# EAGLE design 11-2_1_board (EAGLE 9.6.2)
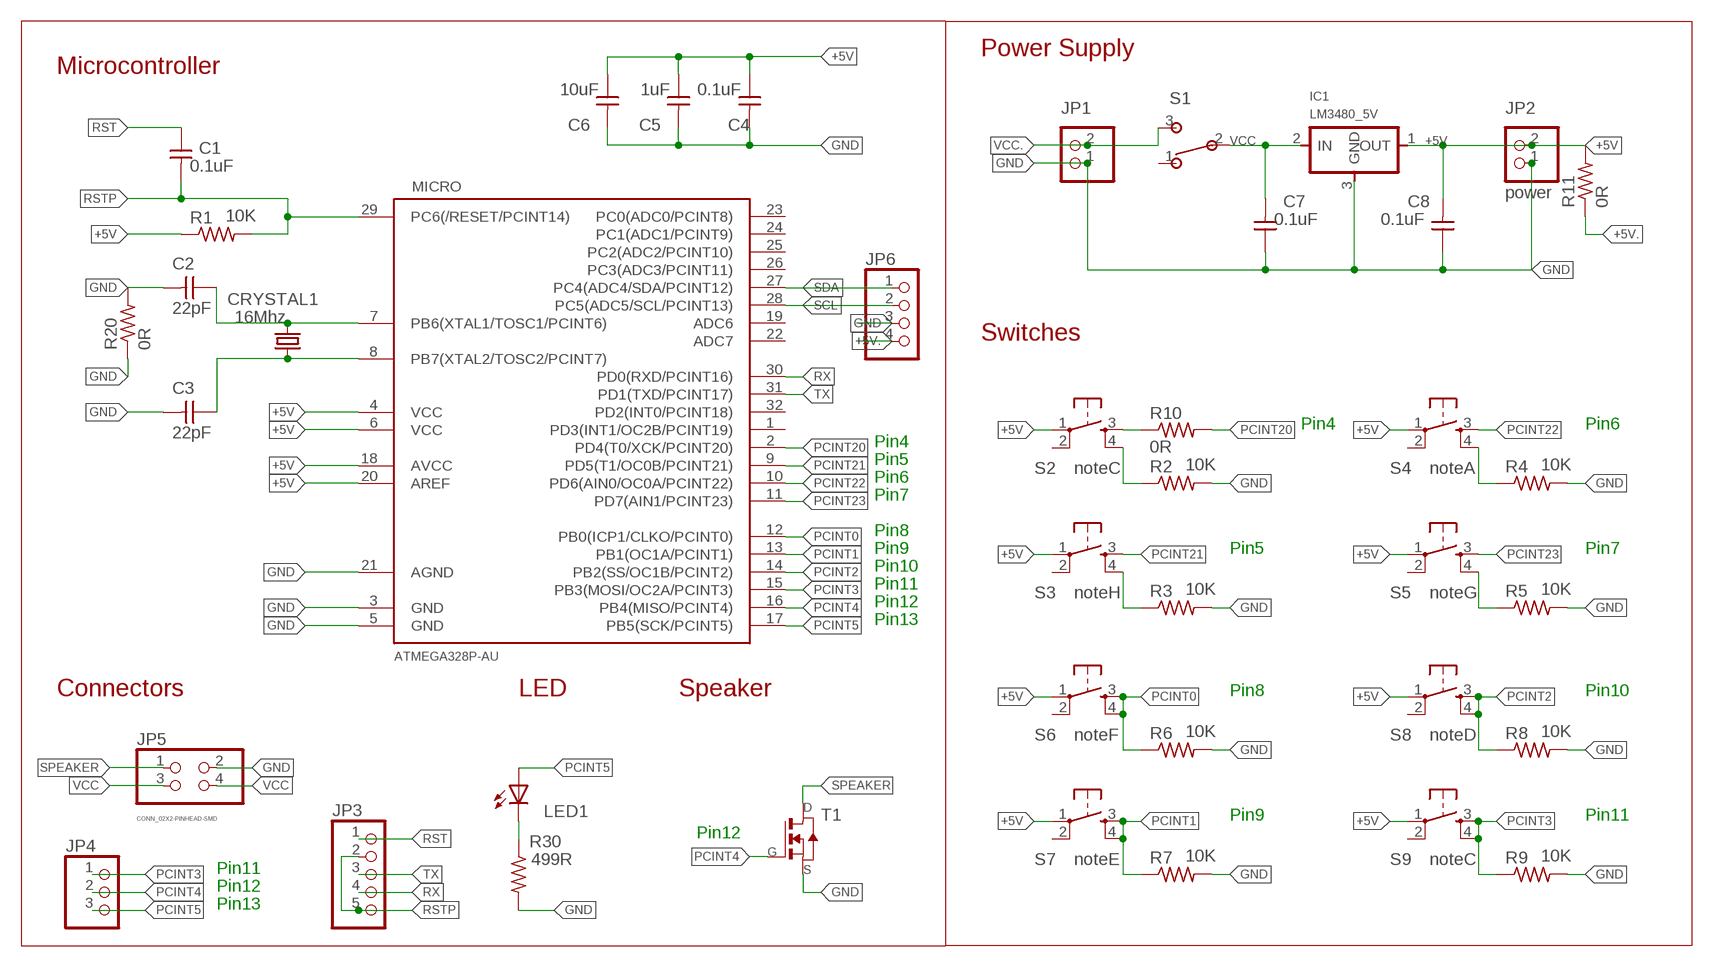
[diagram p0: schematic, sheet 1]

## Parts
C1  0.1uF  CAP_UNPOLARIZEDFAB  [C1206FAB]
C2  22pF  CAP_UNPOLARIZEDFAB  [C1206FAB]
C3  22pF  CAP_UNPOLARIZEDFAB  [C1206FAB]
C4  0.1uF  CAP_UNPOLARIZEDFAB  [C1206FAB]
C5  1uF  CAP_UNPOLARIZEDFAB  [C1206FAB]
C6  10uF  CAP_UNPOLARIZEDFAB  [C1206FAB]
C7  0.1uF  CAP_UNPOLARIZEDFAB  [C1206FAB]
C8  0.1uF  CAP_UNPOLARIZEDFAB  [C1206FAB]
CRYSTAL1  16Mhz  CSM-7X-DU  [CSM-7X-DU]
IC1  LM3480_5V  VR_REGULATOR-SOT23SOT23  [SOT23]
JP1  PINHD-1X2  [1X02]
JP2  power  PINHD-1X2  [1X02]
JP3  PINHD-1X5  [1X05]
JP4  .  PINHD-1X3  [1X03]
JP5  CONN_02X2-PINHEAD-SMD  [2X02SMD]
JP6  PINHD-1X4  [1X04]
LED1  LEDFAB1206  [LED1206FAB]
MICRO  ATMEGA328P-AU  ATMEGA48/88/168-AU  [TQFP32-08]
R1  10K  R1206FAB  [R1206FAB]
R2  10K  R1206FAB  [R1206FAB]
R3  10K  R1206FAB  [R1206FAB]
R4  10K  R1206FAB  [R1206FAB]
R5  10K  R1206FAB  [R1206FAB]
R6  10K  R1206FAB  [R1206FAB]
R7  10K  R1206FAB  [R1206FAB]
R8  10K  R1206FAB  [R1206FAB]
R9  10K  R1206FAB  [R1206FAB]
R10  0R  R1206FAB  [R1206FAB]
R11  0R  R1206FAB  [R1206FAB]
R20  0R  R1206FAB  [R1206FAB]
R30  499R  R1206FAB  [R1206FAB]
S1  SW_SLIDE-SWITCH  [AYZ0102AGRLC]
S2  noteC  SW_SWITCH_TACTILE_6MM6MM_SWITCH  [6MM_SWITCH]
S3  noteH  SW_SWITCH_TACTILE_6MM6MM_SWITCH  [6MM_SWITCH]
S4  noteA  SW_SWITCH_TACTILE_6MM6MM_SWITCH  [6MM_SWITCH]
S5  noteG  SW_SWITCH_TACTILE_6MM6MM_SWITCH  [6MM_SWITCH]
S6  noteF  SW_SWITCH_TACTILE_6MM6MM_SWITCH  [6MM_SWITCH]
S7  noteE  SW_SWITCH_TACTILE_6MM6MM_SWITCH  [6MM_SWITCH]
S8  noteD  SW_SWITCH_TACTILE_6MM6MM_SWITCH  [6MM_SWITCH]
S9  noteC  SW_SWITCH_TACTILE_6MM6MM_SWITCH  [6MM_SWITCH]
T1  MOSFET_NSOT23  [SOT-23]

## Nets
+5V: C4.1 C5.1 C6.1 C8.2 IC1.1(OUT) JP2.2 MICRO.4(VCC) MICRO.6(VCC) MICRO.18(AVCC) MICRO.20(AREF) R1.1 R11.2 S2.1(P) S3.1(P) S4.1(P) S5.1(P) S6.1(P) S7.1(P) S8.1(P) S9.1(P)
+5V.: JP6.4 R11.1
GND: C2.2 C3.2 C4.2 C5.2 C6.2 C7.1 C8.1 IC1.3(GND) JP1.1 JP2.1 JP5.2 JP6.3 MICRO.3(GND) MICRO.5(GND) MICRO.21(AGND) R2.2 R3.2 R4.2 R5.2 R6.2 R7.2 R8.2 R9.2 R20.1 R20.2 R30.2 T1.2(S)
N$1: LED1.2(C) R30.1
N$2: C2.1 CRYSTAL1.2 MICRO.7(PB6(XTAL1/TOSC1/PCINT6))
N$9: C3.1 CRYSTAL1.1 MICRO.8(PB7(XTAL2/TOSC2/PCINT7))
PCINT0: MICRO.12(PB0(ICP1/CLKO/PCINT0)) R6.1 S6.3(S) S6.4(S1)
PCINT1: MICRO.13(PB1(OC1A/PCINT1)) R7.1 S7.3(S) S7.4(S1)
PCINT2: MICRO.14(PB2(SS/OC1B/PCINT2)) R8.1 S8.3(S) S8.4(S1)
PCINT3: JP4.1 MICRO.15(PB3(MOSI/OC2A/PCINT3)) R9.1 S9.3(S) S9.4(S1)
PCINT4: JP4.2 MICRO.16(PB4(MISO/PCINT4)) T1.3(G)
PCINT5: JP4.3 LED1.1(A) MICRO.17(PB5(SCK/PCINT5))
PCINT20: MICRO.2(PD4(T0/XCK/PCINT20)) R10.2
PCINT20.: R10.1 S2.3(S)
PCINT20..: R2.1 S2.4(S1)
PCINT21: MICRO.9(PD5(T1/OC0B/PCINT21)) S3.3(S)
PCINT21.: R3.1 S3.4(S1)
PCINT22: MICRO.10(PD6(AIN0/OC0A/PCINT22)) S4.3(S)
PCINT22.: R4.1 S4.4(S1)
PCINT23: MICRO.11(PD7(AIN1/PCINT23)) S5.3(S)
PCINT23.: R5.1 S5.4(S1)
RST: C1.1 JP3.1
RSTP: C1.2 JP3.2 JP3.5 MICRO.29(PC6(/RESET/PCINT14)) R1.2
RX: JP3.4 MICRO.30(PD0(RXD/PCINT16))
SCL: JP6.2 MICRO.28(PC5(ADC5/SCL/PCINT13))
SDA: JP6.1 MICRO.27(PC4(ADC4/SDA/PCINT12))
SPEAKER: JP5.1 T1.1(D)
TX: JP3.3 MICRO.31(PD1(TXD/PCINT17))
VCC: C7.2 IC1.2(IN) JP5.3 JP5.4 S1.2
VCC.: JP1.2 S1.3
Unconnected: MICRO.1(PD3(INT1/OC2B/PCINT19)) MICRO.19(ADC6) MICRO.22(ADC7) MICRO.23(PC0(ADC0/PCINT8)) MICRO.24(PC1(ADC1/PCINT9)) MICRO.25(PC2(ADC2/PCINT10)) MICRO.26(PC3(ADC3/PCINT11)) MICRO.32(PD2(INT0/PCINT18)) S1.1 S2.2(P1) S3.2(P1) S4.2(P1) S5.2(P1) S6.2(P1) S7.2(P1) S8.2(P1) S9.2(P1)

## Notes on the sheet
- Power Supply
- Microcontroller
- Switches
- Pin4 | Pin6
- Pin4
- Pin5
- Pin6
- Pin7
- Pin8
- Pin9 | Pin5 | Pin7
- Pin10
- Pin11
- Pin12
- Pin13
- Connectors | LED | Speaker | Pin8 | Pin10
- Pin9 | Pin11
- Pin12
- Pin11
- Pin12
- Pin13

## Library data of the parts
C1-C8 = fab:CAP_UNPOLARIZED
CRYSTAL1 = 01_FAB_Hello:CSM-7X-DU: SMD CRYSTAL; OC_FARNELL: unknown; OC_NEWARK: unknown
IC1 = fab:VR_REGULATOR-SOT23
JP1 JP2 = pinhead:PINHD-1X2: PIN HEADER
JP3 = pinhead:PINHD-1X5: PIN HEADER
JP4 = pinhead:PINHD-1X3: PIN HEADER
JP5 = fab:CONN_02X2-PINHEAD-SMD
JP6 = pinhead:PINHD-1X4: PIN HEADER
LED1 = fab:LED: LED
MICRO = atmega8:ATMEGA48/88/168
R1-R11 R20 R30 = fab:R: Resistor (US Symbol)
S1 = fab:SW_SLIDE-SWITCH: SMD slide-switch AYZ0102AGRLC as found in the fablab inventory. Includes the mounting holes. Made by Zaerc.
S2-S9 = fab:SW_SWITCH_TACTILE_6MM: OMRON SWITCH
T1 = fab:MOSFET_N: MOS FET

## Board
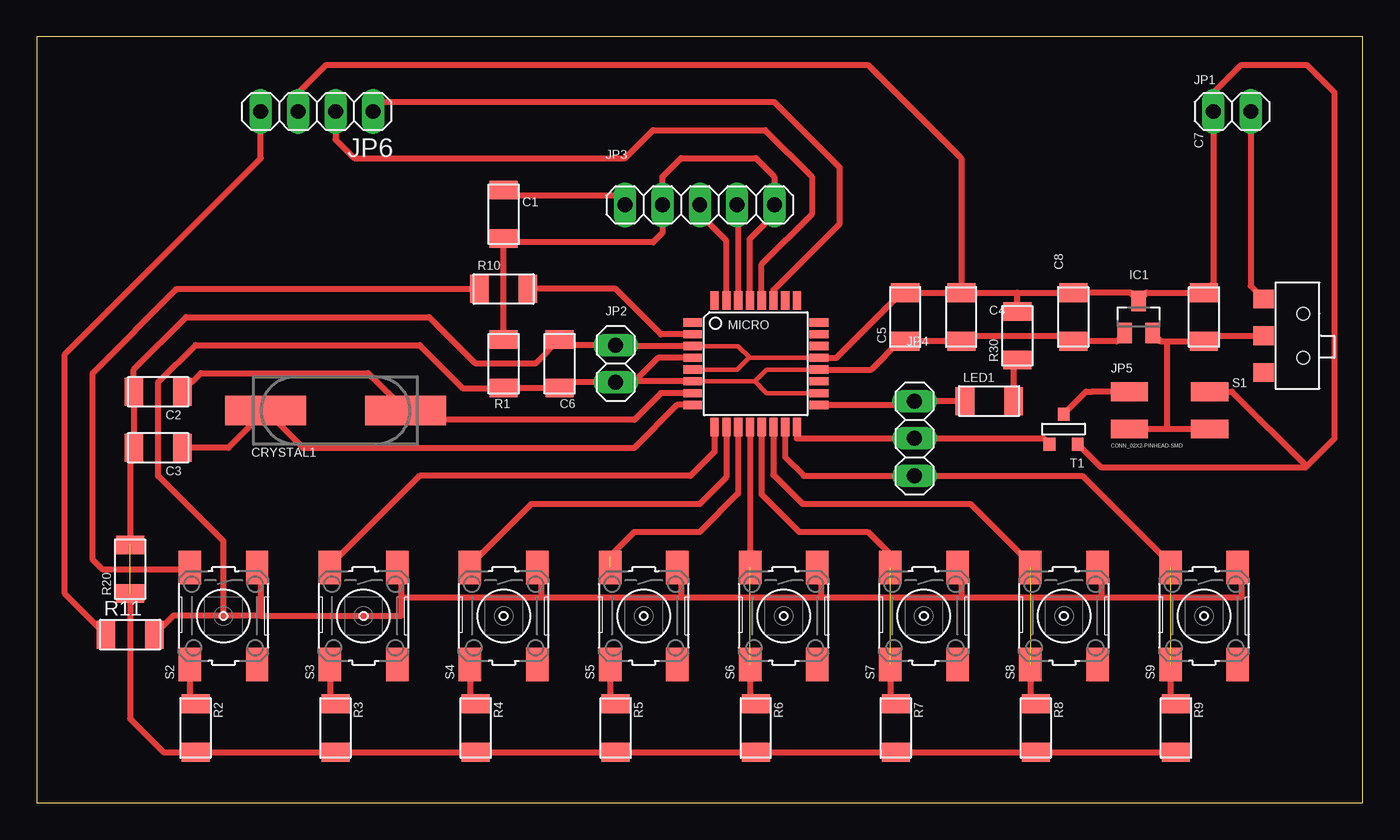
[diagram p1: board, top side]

Size 90.17 x 52.07 mm. Coordinates in mm from the lower left corner, seen from the top.
Outline: 0,0 90.17,0 90.17,52.07 0,52.07 0,0
Copper layers (1*16): Top 0.035mm / dielectric 1.5mm / Bottom 0.035mm
Design rules "default": minimum track width 6mil, minimum drill 0.35mm, track to track 6mil, track to pad 6mil, pad to pad 6mil, via to via 6mil, smd to smd 6mil, copper to edge 40mil, drill to drill 6mil, minimum pad ring 10mil, minimum via ring 8mil, stop-mask expansion 4mil, vias tented up to drill 0mil, thermal gap 10mil
tKeepout: area 21,23.5 to 31.1,33.7; area 19.7,31.1 to 22.2,33; area 29.8,31.1 to 32.4,33; area 29.8,26.7 to 32.4,28.6; area 19.7,26.7 to 22.2,28.6

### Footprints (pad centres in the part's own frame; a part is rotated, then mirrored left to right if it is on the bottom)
C1206FAB = smd 1.27 x 1.905: 1 -1.651,0; 2 1.651,0
CSM-7X-DU = smd 5.5 x 2: 1 -4.75,0; 2 4.75,0
SOT23 = smd 1 x 1.4: 1 -0.95,-1.1; 2 0.95,-1.1; 3 0,1.1
1X02 = drill 1.016 long: 1 -1.27,0; 2 1.27,0
1X05 = drill 1.016 long: 1 -5.08,0; 2 -2.54,0; 3 0,0; 4 2.54,0; 5 5.08,0
1X03 = drill 1.016 long: 1 -2.54,0; 2 0,0; 3 2.54,0
2X02SMD = smd 2.54 x 1.27: 1 -2.54,1.27; 2 2.92,1.27; 3 -2.54,-1.27; 4 2.92,-1.27
1X04 = drill 1.016 long: 1 -3.81,0; 2 -1.27,0; 3 1.27,0; 4 3.81,0
LED1206FAB = smd 1.27 x 1.905: 1 -1.651,0; 2 1.651,0
TQFP32-08 = smd 1.27 x 0.559: 1 -4.293,2.8; 2 -4.293,2; 3 -4.293,1.2; 4 -4.293,0.4; 5 -4.293,-0.4; 6 -4.293,-1.2; 7 -4.293,-2; 8 -4.293,-2.8; 17 4.293,-2.8; 18 4.293,-2; 19 4.293,-1.2; 20 4.293,-0.4; 21 4.293,0.4; 22 4.293,1.2; 23 4.293,2; 24 4.293,2.8 | smd 0.559 x 1.27: 9 -2.8,-4.293; 10 -2,-4.293; 11 -1.2,-4.293; 12 -0.4,-4.293; 13 0.4,-4.293; 14 1.2,-4.293; 15 2,-4.293; 16 2.8,-4.293; 25 2.8,4.293; 26 2,4.293; 27 1.2,4.293; 28 0.4,4.293; 29 -0.4,4.293; 30 -1.2,4.293; 31 -2,4.293; 32 -2.8,4.293
R1206FAB = smd 1.27 x 1.905: 1 -1.651,0; 2 1.651,0
AYZ0102AGRLC = smd 1.27 x 1.397: 1 2.5,-2.3; 2 0,-2.3; 3 -2.5,-2.3 | hole 0.85: -1.5,0.4; 1.5,0.4
6MM_SWITCH = smd 2.286 x 1.524: 1 -3.302,2.286; 2 3.302,2.286; 3 -3.302,-2.286; 4 3.302,-2.286
SOT-23 = smd 0.787 x 0.889: 1 0.025,-1.016; 2 -0.94,1.016; 3 0.991,1.016

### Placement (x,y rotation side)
C1  31.75,40.01 270 top
C2  8.25,27.94 180 top
C3  8.25,24.13 180 top
C4  62.87,33.02 90 top
C5  59.05,33.02 90 top
C6  35.56,29.84 90 top
C7  79.38,33.02 270 top
C8  70.48,33.02 270 top
CRYSTAL1  20.32,26.67 0 top
IC1  74.93,33.02 0 top
JP1  81.28,46.99 0 top
JP2  39.37,29.84 270 top
JP3  45.09,40.64 0 top
JP4  59.69,24.77 90 top
JP5  76.84,26.67 0 top
JP6  19.05,46.99 180 top
LED1  64.77,27.3 0 top
MICRO  48.89,29.84 0 top
R1  31.75,29.84 90 top
R2  10.8,5.08 270 top
R3  20.32,5.08 270 top
R4  29.84,5.08 270 top
R5  39.37,5.08 270 top
R6  48.89,5.08 270 top
R7  58.42,5.08 270 top
R8  67.95,5.08 270 top
R9  77.47,5.08 270 top
R10  31.75,34.92 0 top
R11  6.35,11.43 0 top
R20  6.35,15.88 90 top
R30  66.68,31.75 90 top
S1  85.73,31.75 270 top
S2  12.7,12.7 270 top
S3  22.22,12.7 270 top
S4  31.75,12.7 270 top
S5  41.27,12.7 270 top
S6  50.8,12.7 270 top
S7  60.32,12.7 270 top
S8  69.85,12.7 270 top
S9  79.38,12.7 270 top
T1  69.85,25.4 180 top

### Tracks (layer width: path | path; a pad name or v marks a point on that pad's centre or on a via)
+5V
  Top 0.305: 48.82,28.64 49.62,27.84 MICRO.18 | MICRO.20 49.62,29.45 48.82,28.64 | 48.82,28.64 MICRO.6
  Top 0.406: 15.24,12.7 12.7,12.7 | 15.24,12.7 24.77,12.7 24.77,13.97 | S2.1 15.24,15.75 15.24,12.7 | S3.1 24.77,15.75 24.77,13.97 | 24.77,13.97 34.29,13.97 | S4.1 34.29,15.75 34.29,13.97 | 34.29,13.97 43.81,13.97 | 43.81,13.97 53.34,13.97 | 53.34,13.97 62.87,13.97 | S5.1 43.81,15.75 43.81,13.97 | S6.1 53.34,15.75 53.34,13.97 | S7.1 62.87,15.75 62.87,13.97 | 62.87,13.97 72.39,13.97 | S8.1 72.39,15.75 72.39,13.97 | 72.39,13.97 81.92,13.97 81.92,15.75 S9.1 | MICRO.6 40.64,28.64 | 40.64,28.64 39.44,28.64 JP2.2 35.56,28.57 C6.1 R1.1 28.96,28.19 26.04,31.11 10.8,31.11 8.25,28.57 8.25,22.23 12.7,17.78 12.7,12.7 | MICRO.20 56.75,29.45 58.67,31.37 C5.1 C4.1 63.25,31.75 70.1,31.75 C8.2 73.43,31.37 IC1.1 | 12.7,12.7 9.27,12.7 R11.2 | MICRO.4 42.24,30.25 40.64,28.64
+5V.
  Top 0.406: R11.1 1.91,14.22 1.91,30.48 15.24,43.81 JP6.4
GND  (1 unrouted)
  Top 0.305: MICRO.21 48.49,30.25 | 48.49,30.25 47.7,31.05 MICRO.3 | MICRO.5 47.62,29.45 48.42,30.25 48.49,30.25
  Top 0.406: R20.1 6.35,5.71 8.64,3.43 R2.2 R3.2 R4.2 R5.2 R6.2 | R6.2 53.72,3.43 | 49.15,3.17 R6.2 | R6.2 R7.2 R8.2 R9.2 77.72,3.17 | C6.2 35.56,31.11 | MICRO.3 39.44,31.05 JP2.1 35.94,31.11 C6.2 | C6.2 33.91,29.84 29.84,29.84 26.67,33.02 10.16,33.02 6.6,29.46 C2.2 C3.2 6.35,23.88 R20.2 | C4.2 66.68,34.67 | C4.2 62.87,43.81 56.52,50.16 19.68,50.16 17.78,48.26 JP6.3 | MICRO.21 54.38,30.25 58.8,34.67 C5.2 C4.2 | 70.87,34.29 C8.1 | C8.1 74.38,34.67 IC1.3 75.48,34.67 C7.1 80.01,35.31 JP1.1 80.01,48.26 81.92,50.16 86.36,50.16 88.27,48.26 88.27,24.77 86.36,22.86 | 66.68,34.67 C8.1 | R30.2 66.68,34.67 | T1.2 72.35,22.82 86.32,22.82 86.36,22.86 | JP5.2 81.28,27.94 86.36,22.86
N$1
  Top 0.406: R30.1 66.42,29.84 LED1.2
N$2
  Top 0.406: MICRO.7 42.45,27.84 40.64,26.04 25.7,26.04 CRYSTAL1.2 22.53,29.21 11.18,29.21 C2.1
N$9
  Top 0.406: MICRO.8 43.55,27.05 40.64,24.13 18.11,24.13 CRYSTAL1.1 13.03,24.13 C3.1
PCINT0  (1 unrouted)
  Top 0.406: S6.4 48.51,7.37 49.53,6.35 49.28,6.35 R6.1 | MICRO.12 48.49,16.02 S6.3
PCINT1  (1 unrouted)
  Top 0.406: S7.4 58.04,7.11 R7.1 | MICRO.13 49.3,20.95 51.84,18.41 56.52,18.41 58.04,16.89 S7.3 57.78,16.26
PCINT2  (1 unrouted)
  Top 0.406: S8.4 67.56,7.11 R8.1 | 50.16,25.48 MICRO.14 50.09,22.3 52.07,20.32 63.5,20.32 67.56,16.26 S8.3
PCINT3  (1 unrouted)
  Top 0.406: S9.4 77.09,7.11 R9.1 | MICRO.15 50.89,23.5 52.16,22.23 JP4.1 71.12,22.23 77.09,16.26 S9.3
PCINT4
  Top 0.406: MICRO.16 51.7,24.77 JP4.2 68.48,24.77 T1.3
PCINT5
  Top 0.406: MICRO.17 59.43,27.05 JP4.3 LED1.1
PCINT20
  Top 0.406: MICRO.2 42.45,31.84 39.37,34.92 R10.2
PCINT20.
  Top 0.406: S2.3 10.29,15.88 4.45,15.88 3.81,16.51 3.81,29.21 9.53,34.92 R10.1
PCINT20..
  Top 0.406: S2.4 10.41,7.11 R2.1
PCINT21
  Top 0.406: S3.3 19.94,16.13 26.04,22.23 44.45,22.23 46.09,23.87 MICRO.9
PCINT21.
  Top 0.406: S3.4 19.94,7.11 R3.1
PCINT22
  Top 0.406: MICRO.10 46.89,22.13 45.09,20.32 33.66,20.32 29.46,16.13 S4.3
PCINT22.
  Top 0.406: S4.4 29.46,7.11 R4.1
PCINT23  (1 unrouted)
  Top 0.406: MICRO.11 47.7,21.02 45.09,18.41 40.64,18.41 38.99,16.76
PCINT23.
  Top 0.406: S5.4 38.99,7.11 R5.1
RST
  Top 0.406: JP3.1 39.37,41.27 32.13,41.27 C1.1
RSTP
  Top 0.406: R1.2 31.75,38.1 | 31.75,38.1 C1.2 | 31.75,38.1 41.91,38.1 42.55,38.73 JP3.2 42.55,42.55 43.81,43.81 48.89,43.81 50.16,42.55 JP3.5 50.16,40.01 48.49,38.34 MICRO.29
RX
  Top 0.406: JP3.4 47.7,40.57 MICRO.30
SCL
  Top 0.406: MICRO.28 49.3,36.59 52.7,40.01 52.7,42.55 49.53,45.72 41.91,45.72 40.01,43.81 21.59,43.81 20.32,45.09 JP6.2
SDA
  Top 0.406: MICRO.27 50.09,34.85 54.61,39.37 54.61,43.18 50.16,47.62 23.49,47.62 JP6.1
SPEAKER
  Top 0.406: JP5.1 71.76,27.94 71.35,27.94 T1.1
TX
  Top 0.406: JP3.3 45.09,40.01 46.89,38.2 MICRO.31
VCC
  Top 0.406: IC1.2 76.43,31.37 76.84,31.37 | JP5.4 76.84,25.4 | 76.84,25.4 JP5.3 | 76.84,31.37 C7.2 79.76,31.75 S1.2 | 76.84,31.37 76.84,25.4
VCC.
  Top 0.406: JP1.2 82.55,35.12 S1.3

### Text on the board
tTest: RST | TX | RX | RSTP | GND | 5V | P13 | P12 | P11
Measures: OLED 0,96" / 28,5x28 mm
